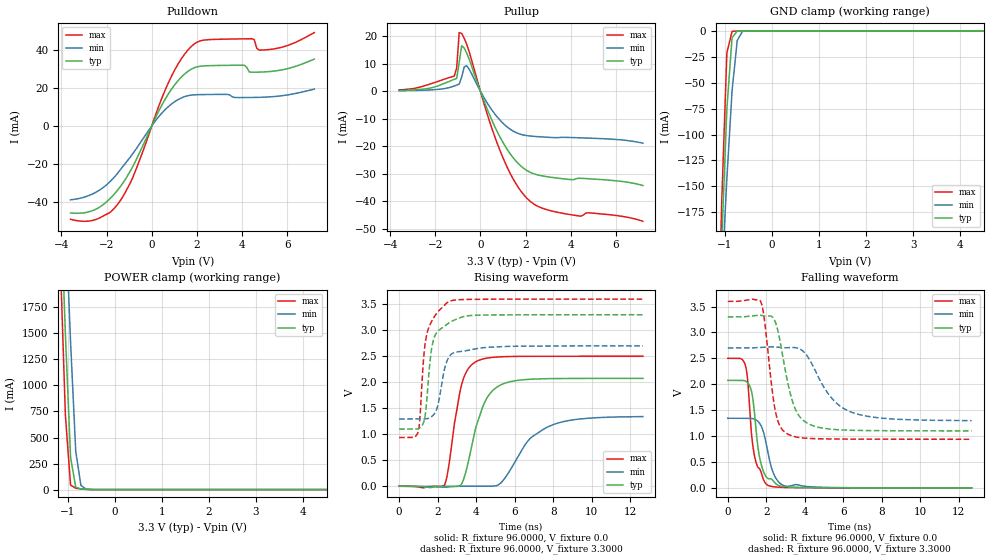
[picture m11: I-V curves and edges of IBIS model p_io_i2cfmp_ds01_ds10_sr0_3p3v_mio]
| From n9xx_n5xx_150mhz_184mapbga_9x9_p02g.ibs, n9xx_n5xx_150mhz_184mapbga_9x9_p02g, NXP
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[Model] p_io_i2cfmp_ds01_ds10_sr0_3p3v_mio
|   Model p_io_i2cfmp_ds01_ds10_sr0_3p3v_mio
| This model was characterised for following simulation conditions:
| External (pad) voltage:
|   - Typ: 3.3V,   - Min: 2.7V,   - Max: 3.6V
| Library cells for typ/min/max conditions are connected as defined below:
|  pad - External Pad
|  ipp_do_lv - Core Input
|  ipp_obe_lv - Output Buffer Enable
|  IOGC - NC
|  REFH3V3 - REFH3V3
|  REFL3V3 - REFL3V3
|  ZI - NC
|  abut_ncal_vddio[1] - vddio
|  abut_ncal_vddio[2] - vddio
|  abut_ncal_vddio[3] - vssio
|  abut_ncal_vddio[4] - vddio
|  abut_ncal_vddio[5] - vddio
|  abut_ncal_vddio[6] - vssio
|  abut_pcal_vddio[1] - vssio
|  abut_pcal_vddio[2] - vssio
|  abut_pcal_vddio[3] - vddio
|  abut_pcal_vddio[4] - vssio
|  abut_pcal_vddio[5] - vssio
|  abut_pcal_vddio[6] - vddio
|  ipp_do_1p8v - ipp_do_1p8v
|  ipp_dse_lv[0] - vdd_lv
|  ipp_dse_lv[1] - 0
|  ipp_eftd_lv - NC
|  ipp_ina_mux_vddio - NC
|  ipp_ina_mux_vddio[0] - NC
|  ipp_ina_mux_vddio[1] - NC
|  ipp_ina_r0_vddio - NC
|  ipp_ina_r0a_vddio - NC
|  ipp_ina_r0b_vddio - NC
|  ipp_ina_r0c_vddio - NC
|  ipp_ina_r0d_vddio - NC
|  ipp_ina_r0e_vddio - NC
|  ipp_ina_r0f_vddio - NC
|  ipp_ina_r300_vddio - NC
|  ipp_ina_r300a_vddio - NC
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Model_type I/O
Polarity   Non-Inverting
Enable   Active-High
Vinl =   0.9900V
Vinh =   2.3100V
Vmeas =  1.6500V
Cref =   30.0000pF
Rref =   1.0000M
Vref =   3.3000V
C_comp   1.7403pF   1.7015pF   1.7922pF
|C_comp_pullup   0.6944pF   0.7580pF   0.6573pF
|C_comp_pulldown   0.9326pF   0.9177pF   0.9316pF
[Model Spec]
| variable   typ   min   max
Vinh   2.3100V   1.8900V   2.5200V
Vinl   0.9900V   0.8100V   1.0800V
[Temperature Range]   25.0000   0.1250k   -40.0000
[Voltage Range]   3.3000V   2.7000V   3.6000V
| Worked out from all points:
|   slope of the pulldown table from 0 to 0.495 V, typ, clamps not added: 41.2 ohm
|   slope of the pullup table from 0 to 0.495 V, typ, clamps not added: 48.1 ohm
|   GND clamp passes 1 mA (typ) near -0.75 V on its own axis
|   POWER clamp passes 1 mA (typ) near -0.52 V on its own axis
|   rising waveform, R_fixture 96.0000, V_fixture 0.0: 20-80 % time 946ps typ, 1.7ns min, 658ps max; typ from 0 V to 2.08 V
|   rising waveform, R_fixture 96.0000, V_fixture 3.3000: 20-80 % time 414ps typ, 471ps min, 447ps max; typ from 1.1 V to 3.3 V
|   falling waveform, R_fixture 96.0000, V_fixture 0.0: 20-80 % time 441ps typ, 531ps min, 409ps max; typ from 2.08 V to 0 V
|   falling waveform, R_fixture 96.0000, V_fixture 3.3000: 20-80 % time 784ps typ, 1.51ns min, 514ps max; typ from 3.3 V to 1.1 V
[Pulldown]
|Voltage   I(typ)   I(min)   I(max)
-3.6V     -45.91mA   -38.97mA   -49.24mA
-2.5V     -44.06mA   -35.15mA   -49.44mA
-1.4V     -32.16mA   -23.22mA   -39.53mA
-850mV    -21.66mA   -14.77mA   -27.43mA
800mV     18.06mA    10.83mA    24.4mA
1.35V     26.21mA    14.95mA    36.11mA
1.9V      30.74mA    16.39mA    43.35mA
4.1V      31.97mA    14.95mA    45.9mA
4.43V     28.32mA    14.99mA    45.97mA
4.65V     28.33mA    15.03mA    40.92mA
5.09V     28.54mA    15.22mA    40.14mA
7.2V      35.25mA    19.41mA    49.21mA
[Pullup]
|Voltage   I(typ)   I(min)   I(max)
-3.6V     311.2uA    185.3uA    486.9uA
-1.16V    4.313mA    1.883mA    5.48mA
-1.05V    4.647mA    2.223mA    8.477mA
-940mV    10.46mA    2.573mA    21.3mA
-830mV    16.55mA    5.158mA    20.99mA
-720mV    15.7mA     8.801mA    19.26mA
-610mV    13.89mA    9.254mA    17.11mA
820mV     -15.89mA   -10.08mA   -20.54mA
1.48V     -24.47mA   -14.6mA    -32.29mA
2.03V     -28.65mA   -16.09mA   -38.62mA
3.46V     -31.6mA    -16.83mA   -44.04mA
7.2V      -34.25mA   -18.88mA   -47.24mA
[GND_clamp]
|Voltage   I(typ)   I(min)   I(max)
-3.6V     -4.377A    -3.283A    -5.855A
-1.18V    -351.7mA   -346.5mA   -367.9mA
-1.07V    -204.2mA   -241.2mA   -166.2mA
-960mV    -75.42mA   -142.6mA   -21.4mA
-850mV    -6.575mA   -58.21mA   -529.8uA
-740mV    -281.6uA   -9.383mA   -183.8uA
-630mV    -73.66uA   -605.1uA   -74.76uA
-410mV    -3.148uA   -9.219uA   -1.868uA
7.2V      0A         0A         0A
[POWER_clamp]
|Voltage   I(typ)   I(min)   I(max)
-3.6V     34.56A     31.8A      37.41A
-1.16V    2.902A     3.904A     2.233A
-1.05V    1.495A     2.658A     715.5mA
-940mV    310.6mA    1.419A     44.07mA
-830mV    22.38mA    368.3mA    13.28mA
-720mV    6.713mA    39.84mA    7.005mA
-610mV    2.702mA    5.591mA    2.612mA
7.2V      0A         0A         0A
[Ramp]
| variable   typ   min   max
dV/dt_r  1.2450/0.9465n   0.8039/1.6972n   1.5004/0.6577n
dV/dt_f  1.3202/0.7840n   0.8412/1.5056n   1.5973/0.5143n
R_load = 96.0000
[Rising Waveform]
R_fixture= 96.0000
V_fixture= 0.0
V_fixture_min= 0.0
V_fixture_max= 0.0
|time   V(typ)   V(min)   V(max)
0s        3.929nV    315.7nV    13.68nV
2.358ns   377.1uV    -16.94mV   27.38mV
2.542ns   -457.4uV   -12.83mV   300.6mV
3.256ns   54.03mV    199.3uV    1.967V
4.015ns   1.169V     -1.183mV   2.401V
4.705ns   1.775V     -1.099mV   2.473V
5.672ns   2.003V     251.7mV    2.495V
6.735ns   2.057V     890.2mV    2.5V
7.94ns    2.071V     1.176V     2.501V
12.67ns   2.075V     1.34V      2.501V
[Rising Waveform]
R_fixture= 96.0000
V_fixture= 3.3000
V_fixture_min= 2.7000
V_fixture_max= 3.6000
|time   V(typ)   V(min)   V(max)
0s        1.099V     1.294V     937.7mV
963.5ps   1.104V     1.294V     1.023V
1.07ns    1.122V     1.294V     1.269V
1.279ns   1.236V     1.294V     2.496V
1.44ns    1.67V      1.299V     2.929V
1.61ns    2.427V     1.321V     3.115V
1.774ns   2.801V     1.369V     3.228V
2.547ns   3.133V     2.459V     3.546V
4.661ns   3.296V     2.674V     3.599V
12.67ns   3.3V       2.7V       3.6V
[Falling Waveform]
R_fixture= 96.0000
V_fixture= 0.0
V_fixture_min= 0.0
V_fixture_max= 0.0
|time   V(typ)   V(min)   V(max)
0s        2.075V     1.344V     2.501V
900ps     2.065V     1.343V     2.383V
1.029ns   2.031V     1.344V     2.098V
1.21ns    1.897V     1.342V     1.141V
1.384ns   1.464V     1.327V     628.1mV
1.668ns   562.9mV    1.239V     360.7mV
2.104ns   178mV      651.5mV    46.29mV
2.457ns   93.85mV    215.2mV    18.13mV
3.015ns   20.86mV    32.49mV    7.636mV
12.67ns   7.514uV    76.15uV    1.079uV
[Falling Waveform]
R_fixture= 96.0000
V_fixture= 3.3000
V_fixture_min= 2.7000
V_fixture_max= 3.6000
|time   V(typ)   V(min)   V(max)
0s        3.3V       2.7V       3.6V
1.719ns   3.332V     2.711V     3.589V
1.895ns   3.318V     2.714V     3.281V
2.475ns   3.197V     2.721V     1.477V
3.126ns   2.016V     2.706V     1.036V
3.508ns   1.522V     2.707V     986mV
3.998ns   1.281V     2.607V     960.2mV
5.276ns   1.135V     1.789V     944mV
6.318ns   1.113V     1.477V     941.1mV
12.67ns   1.1V       1.298V     937.9mV
